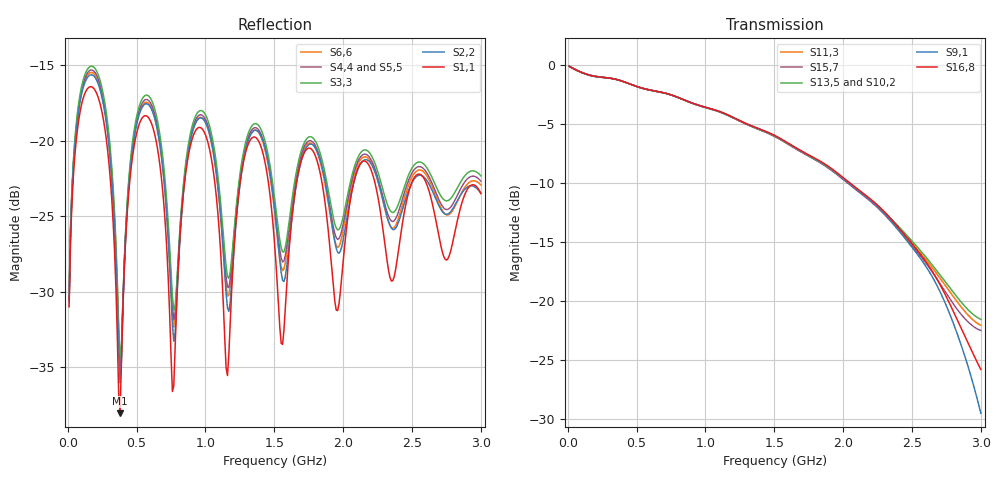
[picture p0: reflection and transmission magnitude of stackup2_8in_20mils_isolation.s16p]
! Touchstone file from project
# GHZ S RI R 50.000000
! Modal data exported
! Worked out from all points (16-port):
!   300 points, 10 MHz to 3 GHz, reference 50 ohm
!   strongest paths, dB at 10 MHz, 760 MHz, 1.51 GHz, 2.26 GHz, 3 GHz:
!     S16,8: -0.1, -2.6, -6.0, -12.0, -25.8
!     S9,1: -0.1, -2.6, -6.0, -12.1, -29.5
!     S13,5: -0.1, -2.6, -6.1, -12.0, -21.5
!     S10,2: -0.1, -2.6, -6.1, -12.1, -20.5
!     S15,7: -0.1, -2.6, -6.1, -12.2, -22.5
!     S11,3: -0.1, -2.6, -6.1, -12.1, -22.0
!   lowest |S11| = -38.1 dB at 380 MHz (marker M1), VSWR 1.03, Z = 51.3 + j0.06 ohm
!   |S11| at or under -10 dB: start of sweep to end of sweep
